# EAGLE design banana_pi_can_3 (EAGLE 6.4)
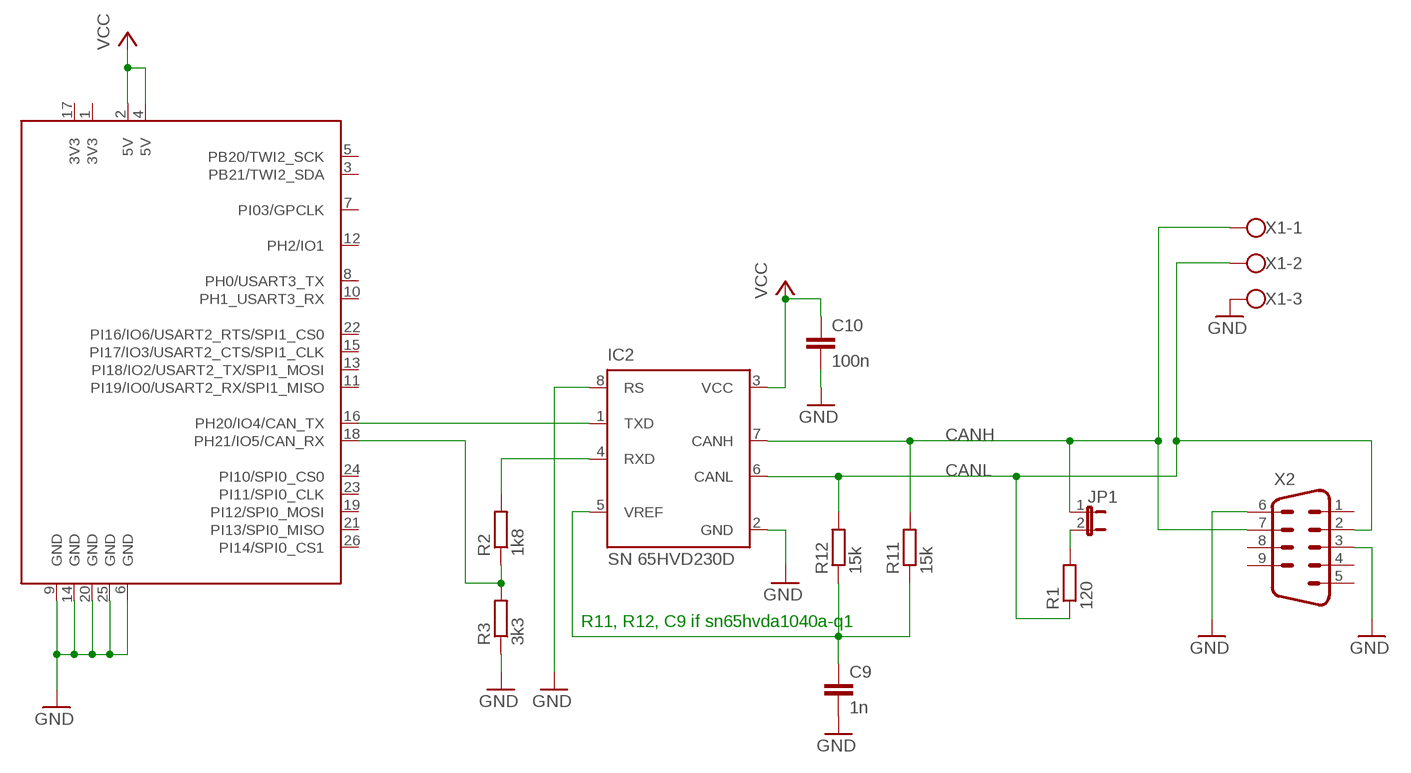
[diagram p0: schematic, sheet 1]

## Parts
C9  1n  C-EUC0805  [C0805]
C10  100n  C-EUC0805  [C0805]
IC2  SN 65HVD230D  PCA82C250T  [SO8]
JP1  JP1E  [JP1]
R1  120  R-EU_R0805  [R0805]
R2  1k8  R-EU_R0805  [R0805]
R3  3k3  R-EU_R0805  [R0805]
R11  15k  R-EU_R0805  [R0805]
R12  15k  R-EU_R0805  [R0805]
U$1  BPI  [BPI_SHIELD]
X1  W237-103  [W237-103]
X2  M09D  [M09D]

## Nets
CANH: IC2.7(CANH) JP1.1 R11.2 X1.1 X2.7
CANL: IC2.6(CANL) R1.1 R12.2 X1.2 X2.2
GND: C9.2 C10.2 IC2.2(GND) IC2.8(RS) R3.1 U$1.6(GND) U$1.9(GND) U$1.14(GND) U$1.20(GND) U$1.25(GND) X1.3 X2.3 X2.6
N$1: IC2.4(RXD) R2.2
N$2: R2.1 R3.2 U$1.18(PH21/IO5/CAN_RX)
N$3: IC2.1(TXD) U$1.16(PH20/IO4/CAN_TX)
N$5: JP1.2 R1.2
N$17: C9.1 IC2.5(VREF) R11.1 R12.1
VCC: C10.1 IC2.3(VCC) U$1.2(5V) U$1.4(5V)
Unconnected: U$1.1(3V3) U$1.3(PB21/TWI2_SDA) U$1.5(PB20/TWI2_SCK) U$1.7(PI03/GPCLK) U$1.8(PH0/USART3_TX) U$1.10(PH1_USART3_RX) U$1.11(PI19/IO0/USART2_RX/SPI1_MISO) U$1.12(PH2/IO1) U$1.13(PI18/IO2/USART2_TX/SPI1_MOSI) U$1.15(PI17/IO3/USART2_CTS/SPI1_CLK) U$1.17(3V3) U$1.19(PI12/SPI0_MOSI) U$1.21(PI13/SPI0_MISO) U$1.22(PI16/IO6/USART2_RTS/SPI1_CS0) U$1.23(PI11/SPI0_CLK) U$1.24(PI10/SPI0_CS0) U$1.26(PI14/SPI0_CS1) X2.1 X2.4 X2.5 X2.8 X2.9

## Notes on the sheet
- R11, R12, C9 if sn65hvda1040a-q1

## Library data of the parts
C9 C10 = rcl:C-EU: CAPACITOR, European symbol
IC2 = micro-philips:PCA82C250: CAN CONTROLLER INTERFACE; OC_FARNELL: 1085275; OC_NEWARK: unknown
JP1 = jumper:JP1E: JUMPER
R1-R3 R11 R12 = rcl:R-EU_: RESISTOR, European symbol
U$1 = bpi_shield:BPI
X1 = con-wago-500:W237-103: WAGO SCREW CLAMP; MPN: 237-103; OC_FARNELL: unknown; OC_NEWARK: 18M7116
X2 = con-subd:M09: SUB-D; OC_FARNELL: unknown; OC_NEWARK: unknown

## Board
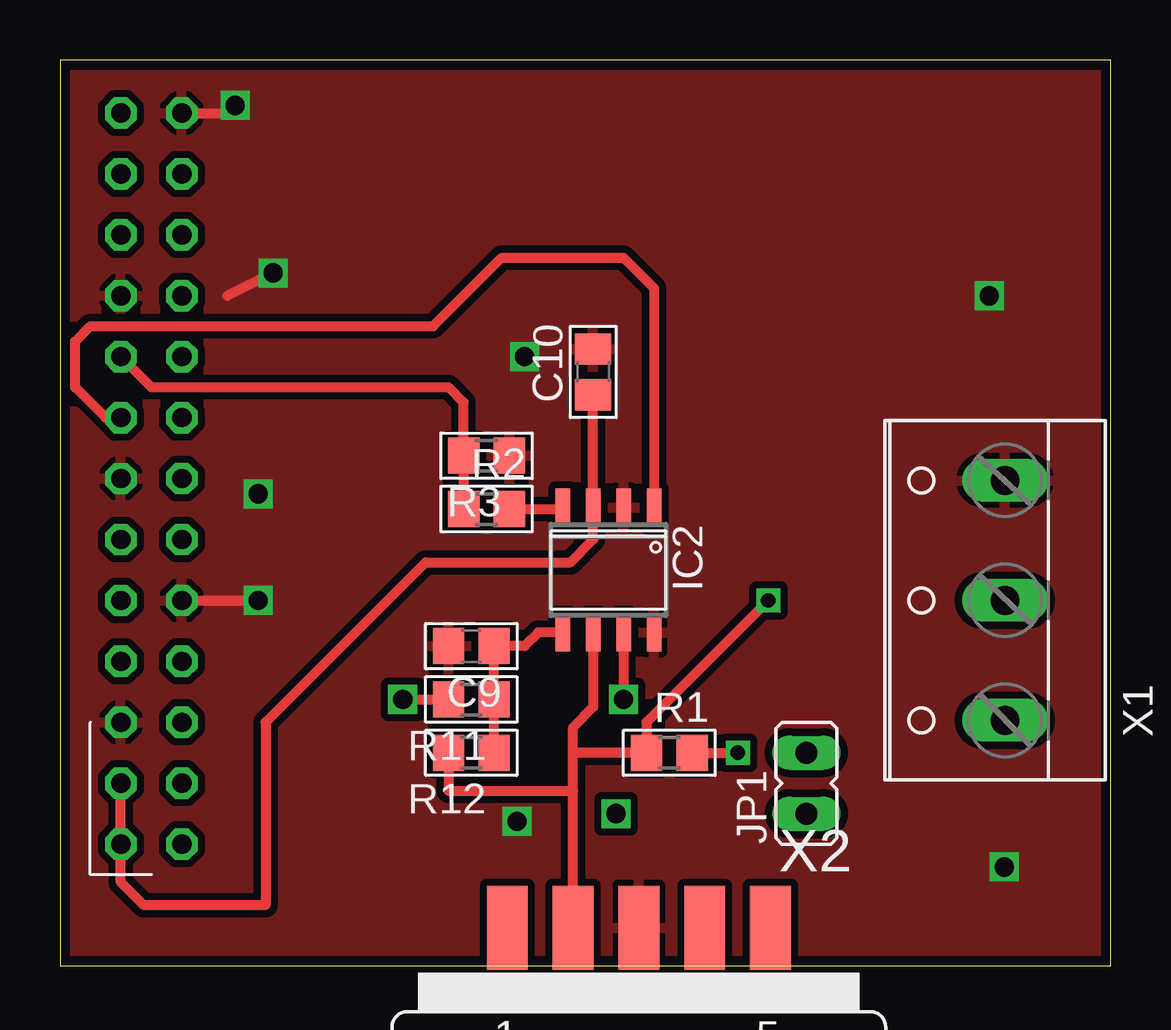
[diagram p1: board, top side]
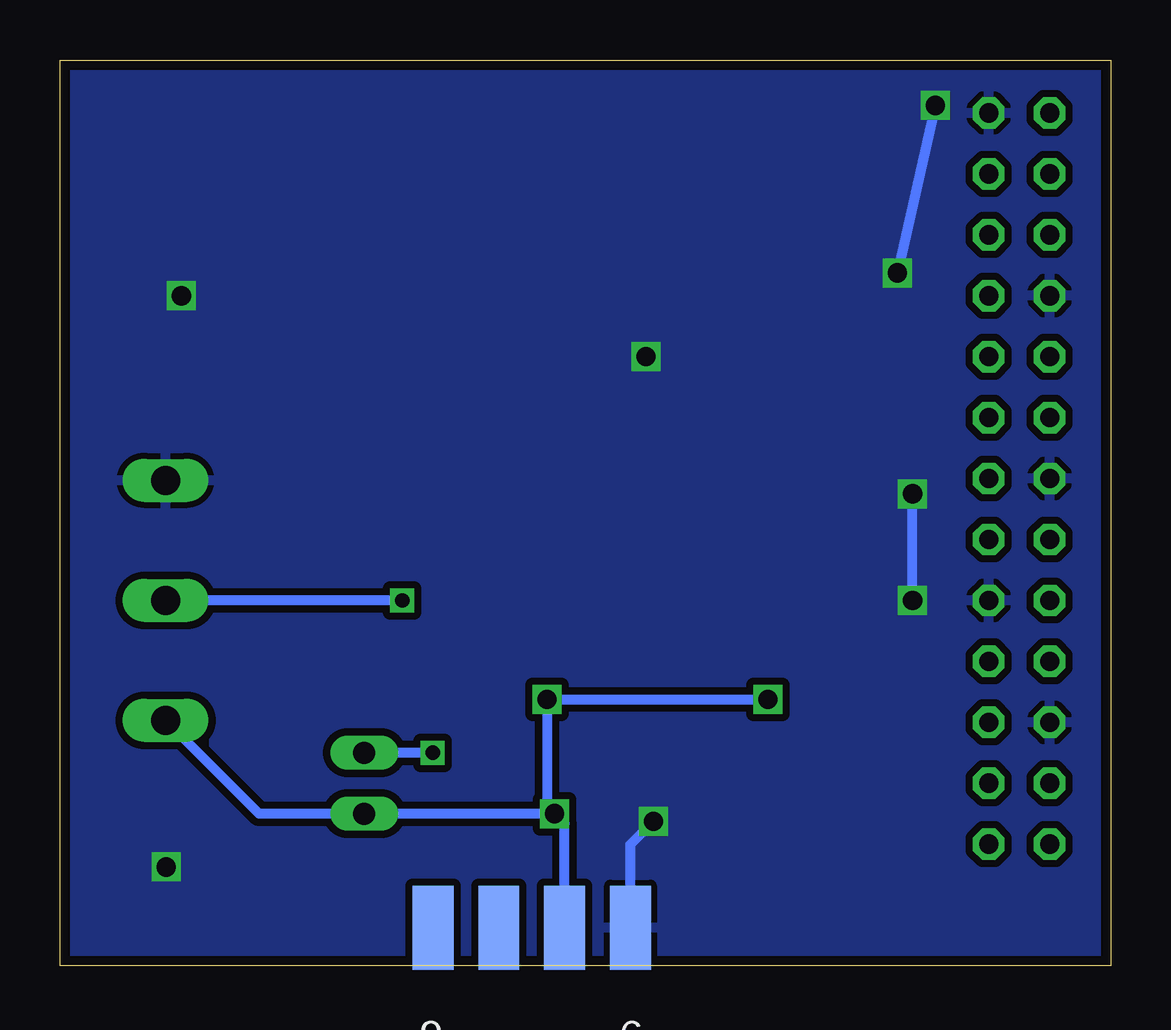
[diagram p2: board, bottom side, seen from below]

Size 43.8 x 37.77 mm. Coordinates in mm from the lower left corner, seen from the top.
Outline: 0,0 43.8,0 43.8,37.77 0,37.77 0,0
Copper layers (1*16): Top 0.035mm / dielectric 1.5mm / Bottom 0.035mm
Design rules "default *": minimum track width 10mil, minimum drill 24mil, track to track 8mil, track to pad 8mil, pad to pad 8mil, via to via 8mil, smd to smd 8mil, copper to edge 16mil, drill to drill 8mil, minimum pad ring 10mil, minimum via ring 8mil, stop-mask expansion 4mil, vias tented up to drill 0mil, thermal gap 10mil

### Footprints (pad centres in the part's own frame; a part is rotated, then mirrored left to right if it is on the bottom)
C0805 = smd 1.3 x 1.5: 1 -0.95,0; 2 0.95,0
SO8 = smd 0.6 x 1.6: 1 -1.905,-2.6; 2 -0.635,-2.6; 3 0.635,-2.6; 4 1.905,-2.6; 5 1.905,2.6; 6 0.635,2.6; 7 -0.635,2.6; 8 -1.905,2.6
JP1 = drill 0.914 long: 1 0,-1.27; 2 0,1.27
R0805 = smd 1.3 x 1.5: 1 -0.95,0; 2 0.95,0
BPI_SHIELD = drill 0.8 octagon: 1 0,0; 2 2.54,0; 3 0,-2.54; 4 2.54,-2.54; 5 0,-5.08; 6 2.54,-5.08; 7 0,-7.62; 8 2.54,-7.62; 9 0,-10.16; 10 2.54,-10.16; 11 0,-12.7; 12 2.54,-12.7; 13 0,-15.24; 14 2.54,-15.24; 15 0,-17.78; 16 2.54,-17.78; 17 0,-20.32; 18 2.54,-20.32; 19 0,-22.86; 20 2.54,-22.86; 21 0,-25.4; 22 2.54,-25.4; 23 0,-27.94; 24 2.54,-27.94; 25 0,-30.48; 26 2.54,-30.48
W237-103 = drill 1.194 long: 1 -5,-1.29; 2 0,-1.29; 3 5,-1.29
M09D = smd 1.7 x 3.5: 1 5.486,-6.045; 2 2.743,-6.045; 3 0,-6.045; 4 -2.743,-6.045; 5 -5.486,-6.045 | smd 1.7 x 3.5 bottom: 6 4.115,-6.045; 7 1.372,-6.045; 8 -1.372,-6.045; 9 -4.115,-6.045

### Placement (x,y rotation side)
C9  17.14,13.34 180 top
C10  22.22,24.76 90 top
IC2  22.86,16.51 180 top
JP1  31.11,7.62 0 top
R1  25.4,8.89 0 top
R2  17.78,19.05 0 top
R3  17.78,21.27 180 top
R11  17.14,11.11 180 top
R12  17.14,8.89 180 top
U$1  5.08,5.08 180 top
X1  38.1,15.24 90 top
X2  24.13,-4.45 180 top

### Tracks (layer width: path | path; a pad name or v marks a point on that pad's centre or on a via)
CANH  (via drill 0.8)
  Top 0.406: IC2.7 v23.5,11.11 | v14.29,11.11 R11.2
  Bottom 0.406: X2.7 22.76,5.93 v23.18,6.35 | v23.18,6.35 23.5,6.67 v23.5,11.11 v14.29,11.11 | v23.18,6.35 JP1.1 35.5,6.35 X1.1
CANL  (via drill 0.6)
  Top 0.406: X2.2 21.39,7.3 | 21.39,7.3 21.39,8.89 | 21.39,8.89 21.39,9.96 22.22,10.79 IC2.6 | 21.39,8.89 R1.1 24.45,10.16 v29.53,15.24 | R12.2 16.2,7.3 16.19,7.3 21.39,7.3
  Bottom 0.406: v29.53,15.24 X1.2
GND  (via drill 0.8)
  Top 0.406: U$1.25 6.98,35.56 v7.3,35.88 | v8.89,28.89 6.98,27.94 | U$1.9 v8.26,15.24
  Bottom 0.406: X2.6 20.02,5.07 v19.05,6.03 | v7.3,35.88 v8.89,28.89 | v8.26,15.24 v8.26,19.68
  other vias: 38.74,27.94 39.37,4.13 19.37,25.4
  pour Top (isolate 0.305): 0,37.78 43.82,37.78 43.82,0 0,0
  pour Bottom (isolate 0.305): -0.32,37.47 44.13,37.47 44.13,0 -0.32,0
N$1
  Top 0.406: R2.2 20.89,19.05 IC2.4
N$2
  Top 0.406: U$1.18 3.81,24.13 16.19,24.13 16.83,23.49 R3.2 R2.1
N$3
  Top 0.406: U$1.16 1.91,22.86 0.64,24.13 0.64,26.04 1.27,26.67 15.56,26.67 18.41,29.53 23.5,29.53 24.77,28.26 IC2.1
N$5  (via drill 0.6)
  Top 0.406: R1.2 v28.26,8.89
  Bottom 0.406: v28.26,8.89 JP1.2
N$17
  Top 0.406: IC2.5 19.94,13.91 19.37,13.34 C9.1 R11.1 R12.1
VCC
  Top 0.406: U$1.4 U$1.2 2.54,3.49 3.49,2.54 8.57,2.54 8.57,10.16 15.24,16.83 21.27,16.83 22.22,17.78 IC2.3 C10.1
